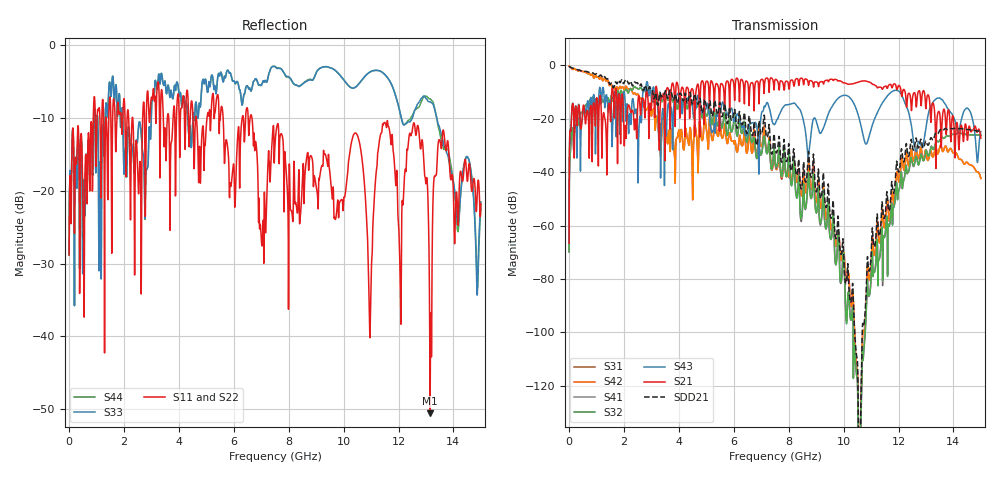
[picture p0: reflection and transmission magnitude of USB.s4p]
! Touchstone generated by fitter/viewer
! HL_PORTMAP 1.0
! PORT  1  (PIN U2.249, Net001, S)
! PORT  2  (PIN U2.248, Net002, S)
! PORT  3  (PIN U3.2, Net047, S)
! PORT  4  (PIN U3.1, Net048, S)
! END_HL_PORTMAP
# HZ S  RI R 5.000000e+001
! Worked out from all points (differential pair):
!   2000 points, 100 kHz to 15 GHz, reference 50 ohm
!   strongest paths, dB at 100 kHz, 3.752 GHz, 7.504 GHz, 11.26 GHz, 15 GHz:
!     S21: -66.6, -6.9, -5.3, -8.2, -27.3
!     S43: -66.6, -21.2, -21.9, -17.1, -24.9
!     S32: -69.9, -13.0, -36.0, -75.4, -26.2
!     S41: -69.9, -13.0, -36.4, -75.1, -26.2
!     S42: -0.3, -24.0, -36.3, -60.8, -42.3
!     S31: -0.3, -24.0, -36.3, -60.9, -42.4
!   taken as a pair (ports 2,1 in; 4,3 out), SDD21 dB: -0.3, -11.2, -30.5, -61.0, -24.9
!   lowest |S11| = -50.6 dB at 13.15 GHz (marker M1), VSWR 1.01, Z = 49.7 + j0.051 ohm
!   |S11| at or under -10 dB: start of sweep to 881.2 MHz; 5.611 GHz to 6.304 GHz (693.3 MHz wide, 11.6 % of centre); 6.662 GHz to end of sweep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
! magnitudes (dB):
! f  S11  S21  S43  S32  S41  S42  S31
! 100 kHz  -28.8  -66.6  -66.6  -69.9  -69.9  -0.3  -0.3
! 810.5 MHz  -10.6  -16.4  -13.1  -14.2  -14.3  -3.7  -3.7
! 4.555 GHz  -17.0  -15.6  -19.0  -12.1  -12.1  -24.0  -24.0
! 8.742 GHz  -16.2  -6.4  -32.1  -43.0  -43.1  -39.2  -38.1
! 10.28 GHz  -13.4  -7.0  -12.7  -95.1  -95.1  -90.4  -90.3
! 13.15 GHz  -50.6  -15.2  -15.9  -32.4  -32.0  -32.6  -32.9
! 15 GHz  -21.8  -27.3  -24.9  -26.2  -26.2  -42.3  -42.4
